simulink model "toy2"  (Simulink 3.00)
settings: Solver=ode45  SolverMode=SingleTasking  StartTime=0.0  StopTime=8000.0  RelTol=1e-3  AbsTol=1e-6

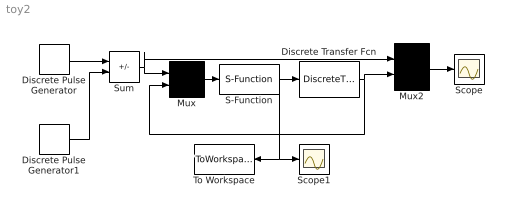
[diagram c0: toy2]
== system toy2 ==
  Discrete Transfer Fcn : DiscreteTransferFcn  Numerator=0.4  Denominator=[1 -.7 .1]  SampleTime=1
  Discrete Pulse Generator : DiscretePulseGenerator  Amplitude=1  Period=90  PulseWidth=30  PhaseDelay=0  SampleTime=1
  Discrete Pulse Generator1 : DiscretePulseGenerator  Amplitude=1  Period=90  PulseWidth=30  PhaseDelay=60  SampleTime=1
  Mux : Mux  Inputs=2
  Mux2 : Mux  Inputs=2
  S-Function : S-Function  FunctionName=toy_ctrl  Parameters=params2  PortCounts=[]  SFunctionModules=''
  Scope : Scope
  Scope1 : Scope
  Sum : Sum  Inputs=+-  SaturateOnIntegerOverflow=on
  To Workspace : ToWorkspace  VariableName=u  SampleTime=-1  SaveFormat=Matrix
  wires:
  Discrete Pulse Generator1/1 -> Sum/2
  Discrete Pulse Generator/1 -> Sum/1
  Sum/1 -> Mux2/1, Mux/1
  S-Function/1 -> Discrete Transfer Fcn/1, Scope1/1, To Workspace/1
  Mux2/1 -> Scope/1
  Discrete Transfer Fcn/1 -> Mux2/2, Mux/2
  Mux/1 -> S-Function/1
